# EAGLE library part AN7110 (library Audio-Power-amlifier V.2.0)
1,2W AUDIO POWER AMPLIFIER
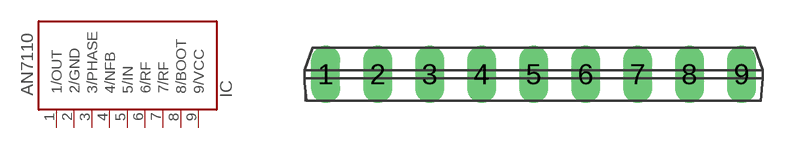
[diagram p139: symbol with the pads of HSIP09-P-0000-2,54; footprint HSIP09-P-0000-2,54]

Designator prefix IC

## AN7110  [HSIP09-P-0000-2,54]
1  1/OUT  out
2  2/GND  pwr
3  3/PHASE
4  4/NFB  in
5  5/IN  in
6  6/RF
7  7/RF
8  8/BOOT
9  9/VCC  pwr

## Footprint HSIP09-P-0000-2,54 (pad centres in mm)
drill 0.9 long: 1 -10.16,0; 2 -7.62,0; 3 -5.08,0; 4 -2.54,0; 5 0,0; 6 2.54,0; 7 5.08,0; 8 7.62,0; 9 10.16,0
